| Teraspeed Modeling Services.
| http://www.teraspeed.com
[IBIS Ver]   3.2
[Comment Char] |_char
[File Name]   lpc1788fet208.ibs
[File Rev]   3.0
[Source]  Measured and created by Teraspeed Consulting Group LLC
[Date]   04-04-2011
[Notes]   Quality Check of this IBIS model: Model Passes IBIS Check
   Model parses into ICX IS. Simulation done with Hyperlynx.
   1. MIN TYP MAX information is based on Temperature and Voltage
   characteristics only.
   2. Package data measured using Tektronix IConnect Software.
[Disclaimer]
| NXP Semiconductors warrants and represents that the IBIS models
| identified herein are owned by NXP Semiconductors (NXP).  The
| models provided are not warranted as fully representing all of the
| operating characteristics and specifications of the semiconductor
| products to which the models relate.  Moreover, unless there is a
| signed, written agreement to the contrary, these models are furnished
| on an "as is" basis without support or warranty of any kind, either
| expressed or implied, regarding the use thereof, and NXP
| specifically disclaims all implied warranties of merchantability and
| fitness of the models for any purpose.
| NXP does not assume any liability arising out of the application
| or use of these IBIS models including infringement of patents and
| copyrights, nor does NXP convey any license under its patents and
| copyrights or the rights of others.
| NXP provides IBIS models as a service to our customers.  You and
| your company shall not distribute, convey, sell, or give these models
| to anyone else without receiving prior written permission from
| NXP.
[Copyright]  NXP Semiconductors 2011. All rights reserved.
|   LPC177x_8x (208 TFBGA package) IBIS Model
|   IBIS Model Created by Teraspeed Consulting Group
|   www.teraspeed.com
[Component] LPC1788FET208
[Manufacturer] NXP Semiconductors
[Package]
| variable   typ   min   max
| TFBGA208
R_pkg  1.000E-02  1.000E-02  1.000E-02
L_pkg  2.355E-09  3.067E-10  4.180E-09
C_pkg  5.803E-13  7.558E-14  1.030E-12
[Pin] signal_name  model_name  R_pin  L_pin C_pin
A1   P3_27   io_pad   1.000E-02  4.180E-09  1.030E-12
A2   VSS   GND   1.000E-02  4.180E-09  1.030E-12
A3   P1_0   io_pad   1.000E-02  3.374E-09  8.314E-13
A4   P4_31   io_pad   1.000E-02  3.027E-09  7.458E-13
A5   P1_4   io_pad   1.000E-02  2.726E-09  6.718E-13
A6   P1_9   io_pad   1.000E-02  2.481E-09  6.113E-13
A7   P1_14   io_pad   1.000E-02  2.298E-09  5.663E-13
A8   P1_15   io_pad   1.000E-02  2.185E-09  5.385E-13
A9   P1_17   io_pad   1.000E-02  2.147E-09  5.291E-13
A10   P1_3   io_pad   1.000E-02  2.185E-09  5.385E-13
A11   P4_15   io_pad   1.000E-02  2.298E-09  5.663E-13
A12   VSS   GND   1.000E-02  4.180E-09  1.030E-12
A13   P3_20   io_pad   1.000E-02  2.726E-09  6.718E-13
A14   P1_11   io_pad   1.000E-02  3.027E-09  7.458E-13
A15   P0_8   io_pad   1.000E-02  3.374E-09  8.314E-13
A16   P1_12   io_pad   1.000E-02  3.761E-09  9.267E-13
A17   P1_5   io_pad   1.000E-02  4.180E-09  1.030E-12
B1   P3_2   io_pad   1.000E-02  3.761E-09  9.267E-13
B2   P3_10   io_pad   1.000E-02  3.312E-09  8.162E-13
B3   P3_1   io_pad   1.000E-02  2.895E-09  7.134E-13
B4   P3_0   io_pad   1.000E-02  2.517E-09  6.201E-13
B5   P1_1   io_pad   1.000E-02  2.185E-09  5.385E-13
B6   VSS   GND   1.000E-02  4.180E-09  1.030E-12
B7   P4_30   io_pad   1.000E-02  1.706E-09  4.203E-13
B8   P4_24   io_pad   1.000E-02  1.577E-09  3.887E-13
B9   P4_25   io_pad   1.000E-02  1.534E-09  3.779E-13
B10   P4_29   io_pad   1.000E-02  1.577E-09  3.887E-13
B11   P1_6   io_pad   1.000E-02  1.706E-09  4.203E-13
B12   P0_4   io_pad   1.000E-02  1.911E-09  4.710E-13
B13   Vdd(3v3)   POWER   1.000E-02  4.180E-09  1.030E-12
B14   P3_19   io_pad   1.000E-02  2.517E-09  6.201E-13
B15   P4_14   io_pad   1.000E-02  2.895E-09  7.134E-13
B16   P4_13   io_pad   1.000E-02  3.312E-09  8.162E-13
B17   P2_0   io_pad   1.000E-02  3.761E-09  9.267E-13
C1   P3_13   io_pad   1.000E-02  3.374E-09  8.314E-13
C2   JTAG_TDI   in_pu   1.000E-02  2.895E-09  7.134E-13
C3   P5_4   io_pad   1.000E-02  2.445E-09  6.024E-13
C4   P0_2   io_pad   1.000E-02  2.031E-09  5.004E-13
C5   P3_9   io_pad   1.000E-02  1.663E-09  4.098E-13
C6   P3_22   io_pad   1.000E-02  1.355E-09  3.338E-13
C7   P1_8   io_pad   1.000E-02  1.119E-09  2.758E-13
C8   P1_10   io_pad   1.000E-02  9.710E-10  2.393E-13
C9   Vdd(3v3)   POWER   1.000E-02  4.180E-09  1.030E-12
C10   P3_21   io_pad   1.000E-02  9.710E-10  2.393E-13
C11   P4_28   io_pad   1.000E-02  1.119E-09  2.758E-13
C12   P0_5   io_pad   1.000E-02  1.355E-09  3.338E-13
C13   P0_7   io_pad   1.000E-02  1.663E-09  4.098E-13
C14   P0_9   io_pad   1.000E-02  2.031E-09  5.004E-13
C15   P3_18   io_pad   1.000E-02  2.445E-09  6.024E-13
C16   P4_12   io_pad   1.000E-02  2.895E-09  7.134E-13
C17   Vdd(3v3)   POWER   1.000E-02  4.180E-09  1.030E-12
D1   JTAG_*TRST   in_pu   1.000E-02  3.027E-09  7.458E-13
D2   P3_28   io_pad   1.000E-02  2.517E-09  6.201E-13
D3   JTAG_TDO   tri_pad   1.000E-02  2.031E-09  5.004E-13
D4   P3_12   io_pad   1.000E-02  1.577E-09  3.887E-13
D5   P3_11   io_pad   1.000E-02  1.168E-09  2.877E-13
D6   P0_3   io_pad   1.000E-02  8.165E-10  2.012E-13
D7   Vdd(3v3)   POWER   1.000E-02  4.180E-09  1.030E-12
D8   P3_8   io_pad   1.000E-02  3.675E-10  9.055E-14
D9   P1_2   io_pad   1.000E-02  3.067E-10  7.558E-14
D10   P1_16   io_pad   1.000E-02  3.675E-10  9.055E-14
D11   Vdd(reg)(3v3) POWER   1.000E-02  4.180E-09  1.030E-12
D12   Vss(reg)   GND   1.000E-02  4.180E-09  1.030E-12
D13   P0_6   io_pad   1.000E-02  1.168E-09  2.877E-13
D14   P1_7   io_pad   1.000E-02  1.577E-09  3.887E-13
D15   P2_2   io_pad   1.000E-02  2.031E-09  5.004E-13
D16   P1_13   io_pad   1.000E-02  2.517E-09  6.201E-13
D17   P2_4   io_pad   1.000E-02  3.027E-09  7.458E-13
E1   P0_26   io_pad   1.000E-02  2.726E-09  6.718E-13
E2   JTAG_TCK   in_tck   1.000E-02  2.185E-09  5.385E-13
E3   JTAG_TMS   in_pu   1.000E-02  1.663E-09  4.098E-13
E4   P3_3   io_pad   1.000E-02  1.168E-09  2.877E-13
E14   P2_1   io_pad   1.000E-02  1.168E-09  2.877E-13
E15   VSS   GND   1.000E-02  4.180E-09  1.030E-12
E16   P2_3   io_pad   1.000E-02  2.185E-09  5.385E-13
E17   P2_6   io_pad   1.000E-02  2.726E-09  6.718E-13
F1   P0_25   io_pad   1.000E-02  2.481E-09  6.113E-13
F2   P3_4   io_pad   1.000E-02  1.911E-09  4.710E-13
F3   P3_29   io_pad   1.000E-02  1.355E-09  3.338E-13
F4   P5_0   io_pad   1.000E-02  8.165E-10  2.012E-13
F14   P4_11   io_pad   1.000E-02  8.165E-10  2.012E-13
F15   P3_17   io_pad   1.000E-02  1.355E-09  3.338E-13
F16   P2_5   io_pad   1.000E-02  1.911E-09  4.710E-13
F17   P3_16   io_pad   1.000E-02  2.481E-09  6.113E-13
G1   P3_5   io_pad   1.000E-02  2.298E-09  5.663E-13
G2   P0_24   io_pad   1.000E-02  1.706E-09  4.203E-13
G3   Vdd(3v3)   POWER   1.000E-02  4.180E-09  1.030E-12
G4   Vdda   POWER   1.000E-02  4.180E-09  1.030E-12
G14   P5_3   od1_pad   1.000E-02  5.430E-10  1.338E-13
G15   P4_27   io_pad   1.000E-02  1.119E-09  2.758E-13
G16   P2_7   io_pad   1.000E-02  1.706E-09  4.203E-13
G17   P4_10   io_pad   1.000E-02  2.298E-09  5.663E-13
H1   P0_23   io_pad   1.000E-02  2.185E-09  5.385E-13
H2   P3_14   io_pad   1.000E-02  1.577E-09  3.887E-13
H3   P3_30   io_pad   1.000E-02  9.710E-10  2.393E-13
H4   Vdd(reg)(3v3) POWER   1.000E-02  4.180E-09  1.030E-12
H14   VSS   GND   1.000E-02  4.180E-09  1.030E-12
H15   P2_8   io_pad   1.000E-02  9.710E-10  2.393E-13
H16   P2_9   io_pad   1.000E-02  1.577E-09  3.887E-13
H17   P4_9   io_pad   1.000E-02  2.185E-09  5.385E-13
J1   P3_6   io_pad   1.000E-02  2.147E-09  5.291E-13
J2   Vssa   GND   1.000E-02  4.180E-09  1.030E-12
J3   P3_31   io_pad   1.000E-02  9.202E-10  2.267E-13
J4   P5_1   io_pad   1.000E-02  3.067E-10  7.558E-14
J14   P0_16   io_pad   1.000E-02  3.067E-10  7.558E-14
J15   P4_23   io_pad   1.000E-02  9.202E-10  2.267E-13
J16   P0_15   io_pad   1.000E-02  1.534E-09  3.779E-13
J17   P4_8   io_pad   1.000E-02  2.147E-09  5.291E-13
K1   VREFP   term   1.000E-02  4.180E-09  1.030E-12
K2   RTCX1   term   1.000E-02  1.577E-09  3.887E-13
K3   *RSTOUT   out_pad   1.000E-02  9.710E-10  2.393E-13
K4   Vss(reg)   GND   1.000E-02  4.180E-09  1.030E-12
K14   P4_22   io_pad   1.000E-02  3.675E-10  9.055E-14
K15   P0_18   io_pad   1.000E-02  9.710E-10  2.393E-13
K16   Vdd(3v3)   POWER   1.000E-02  4.180E-09  1.030E-12
K17   P0_17   io_pad   1.000E-02  2.185E-09  5.385E-13
L1   P3_7   io_pad   1.000E-02  2.298E-09  5.663E-13
L2   RTCX2   term   1.000E-02  1.706E-09  4.203E-13
L3   VSS   GND   1.000E-02  4.180E-09  1.030E-12
L4   P2_30   io_pad   1.000E-02  5.430E-10  1.338E-13
L14   P5_2   od1_pad   1.000E-02  5.430E-10  1.338E-13
L15   P4_26   io_pad   1.000E-02  1.119E-09  2.758E-13
L16   P4_7   io_pad   1.000E-02  1.706E-09  4.203E-13
L17   P0_19   io_pad   1.000E-02  2.298E-09  5.663E-13
M1   P3_15   io_pad   1.000E-02  2.481E-09  6.113E-13
M2   *RESET   in_resetb  1.000E-02  1.911E-09  4.710E-13
M3   Vbat   POWER   1.000E-02  4.180E-09  1.030E-12
M4   XTAL1   term   1.000E-02  8.165E-10  2.012E-13
M14   P4_6   io_pad   1.000E-02  8.165E-10  2.012E-13
M15   P4_21   io_pad   1.000E-02  1.355E-09  3.338E-13
M16   P0_21   io_pad   1.000E-02  1.911E-09  4.710E-13
M17   P0_20   io_pad   1.000E-02  2.481E-09  6.113E-13
N1   RTC_ALARM   rtc_alarm  1.000E-02  2.726E-09  6.718E-13
N2   P2_31   io_pad   1.000E-02  2.185E-09  5.385E-13
N3   P2_29   io_pad   1.000E-02  1.663E-09  4.098E-13
N4   XTAL2   term   1.000E-02  1.168E-09  2.877E-13
N14   P2_12   io_pad   1.000E-02  1.168E-09  2.877E-13
N15   P2_10   io_pad   1.000E-02  1.663E-09  4.098E-13
N16   VSS   GND   1.000E-02  4.180E-09  1.030E-12
N17   P0_22   io_pad   1.000E-02  2.726E-09  6.718E-13
P1   P1_31   io_pad   1.000E-02  3.027E-09  7.458E-13
P2   P1_30   io_pad   1.000E-02  2.517E-09  6.201E-13
P3   P2_27   io_pad   1.000E-02  2.031E-09  5.004E-13
P4   P2_28   io_pad   1.000E-02  1.577E-09  3.887E-13
P5   P2_24   io_pad   1.000E-02  1.168E-09  2.877E-13
P6   Vdd(3v3)   POWER   1.000E-02  4.180E-09  1.030E-12
P7   P1_18   io_pad   1.000E-02  5.430E-10  1.338E-13
P8   Vdd(3v3)   POWER   1.000E-02  4.180E-09  1.030E-12
P9   P1_23   io_pad   1.000E-02  3.067E-10  7.558E-14
P10   Vss(reg)   GND   1.000E-02  4.180E-09  1.030E-12
P11   Vdd(reg)(3v3) POWER   1.000E-02  4.180E-09  1.030E-12
P12   VSS   GND   1.000E-02  4.180E-09  1.030E-12
P13   P2_15   io_pad   1.000E-02  1.168E-09  2.877E-13
P14   P4_17   io_pad   1.000E-02  1.577E-09  3.887E-13
P15   P4_18   io_pad   1.000E-02  2.031E-09  5.004E-13
P16   P4_19   io_pad   1.000E-02  2.517E-09  6.201E-13
P17   Vdd(3v3)   POWER   1.000E-02  4.180E-09  1.030E-12
R1   P0_12   io_pad   1.000E-02  3.374E-09  8.314E-13
R2   P0_13   io_pad   1.000E-02  2.895E-09  7.134E-13
R3   P0_28   od2_pad   1.000E-02  2.445E-09  6.024E-13
R4   P2_25   io_pad   1.000E-02  2.031E-09  5.004E-13
R5   P3_24   io_pad   1.000E-02  1.663E-09  4.098E-13
R6   P0_30   io_pad   1.000E-02  1.355E-09  3.338E-13
R7   P2_19   io_pad   1.000E-02  1.119E-09  2.758E-13
R8   P1_21   io_pad   1.000E-02  9.710E-10  2.393E-13
R9   VSS   GND   1.000E-02  4.180E-09  1.030E-12
R10   P1_26   io_pad   1.000E-02  9.710E-10  2.393E-13
R11   P2_16   io_pad   1.000E-02  1.119E-09  2.758E-13
R12   P2_14   io_pad   1.000E-02  1.355E-09  3.338E-13
R13   P2_17   io_pad   1.000E-02  1.663E-09  4.098E-13
R14   P0_11   io_pad   1.000E-02  2.031E-09  5.004E-13
R15   P4_4   io_pad   1.000E-02  2.445E-09  6.024E-13
R16   P4_5   io_pad   1.000E-02  2.895E-09  7.134E-13
R17   P4_20   io_pad   1.000E-02  3.374E-09  8.314E-13
T1   P0_27   od2_pad   1.000E-02  3.761E-09  9.267E-13
T2   P0_31   io_pad   1.000E-02  3.312E-09  8.162E-13
T3   P3_26   io_pad   1.000E-02  2.895E-09  7.134E-13
T4   P2_26   io_pad   1.000E-02  2.517E-09  6.201E-13
T5   VSS   GND   1.000E-02  4.180E-09  1.030E-12
T6   P3_23   io_pad   1.000E-02  1.911E-09  4.710E-13
T7   P0_14   io_pad   1.000E-02  1.706E-09  4.203E-13
T8   P2_20   io_pad   1.000E-02  1.577E-09  3.887E-13
T9   P1_24   io_pad   1.000E-02  1.534E-09  3.779E-13
T10   P1_25   io_pad   1.000E-02  1.577E-09  3.887E-13
T11   P4_2   io_pad   1.000E-02  1.706E-09  4.203E-13
T12   P1_27   io_pad   1.000E-02  1.911E-09  4.710E-13
T13   P1_28   io_pad   1.000E-02  2.185E-09  5.385E-13
T14   P0_1   io_pad   1.000E-02  2.517E-09  6.201E-13
T15   P0_10   io_pad   1.000E-02  2.895E-09  7.134E-13
T16   P2_13   io_pad   1.000E-02  3.312E-09  8.162E-13
T17   P2_11   io_pad   1.000E-02  3.761E-09  9.267E-13
U1   USB_D2N   io_pad   1.000E-02  4.180E-09  1.030E-12
U2   P3_25   io_pad   1.000E-02  3.761E-09  9.267E-13
U3   P2_18   io_pad   1.000E-02  3.374E-09  8.314E-13
U4   P0_29   io_pad   1.000E-02  3.027E-09  7.458E-13
U5   P2_23   io_pad   1.000E-02  2.726E-09  6.718E-13
U6   P1_19   io_pad   1.000E-02  2.481E-09  6.113E-13
U7   P1_20   io_pad   1.000E-02  2.298E-09  5.663E-13
U8   P1_22   io_pad   1.000E-02  2.185E-09  5.385E-13
U9   P4_0   io_pad   1.000E-02  2.147E-09  5.291E-13
U10   P4_1   io_pad   1.000E-02  2.185E-09  5.385E-13
U11   P2_21   io_pad   1.000E-02  2.298E-09  5.663E-13
U12   P2_22   io_pad   1.000E-02  2.481E-09  6.113E-13
U13   Vdd(3v3)   POWER   1.000E-02  4.180E-09  1.030E-12
U14   P1_29   io_pad   1.000E-02  3.027E-09  7.458E-13
U15   P0_0   io_pad   1.000E-02  3.374E-09  8.314E-13
U16   P4_3   io_pad   1.000E-02  3.761E-09  9.267E-13
U17   P4_16   io_pad   1.000E-02  4.180E-09  1.030E-12
[Model Selector]  in_pu
pu_2.5v   input w/int pull up,vdd=2.5v
pu_3.3v   input w/int pull up,vdd=3.3v
[Model Selector]  in_resetb
reset_2.5v   reset input w/int pull up,vdd=2.5v
reset_3.3v   reset input w/int pull up,vdd=3.3v
[Model Selector]  in_tck
tck_2.5v   tck input,vdd=2.5v
tck_3.3v   tck input,vdd=3.3v
[Model Selector]  io_pad
io_2.5v   io pin,vdd=2.5v
io_3.3v   io pin,vdd=3.3v
io_pd_2.5v  io pin w/int pull dwn,vdd=2.5v
io_pd_3.3v  io pin w/int pull dwn,vdd=3.3v
io_pu_2.5v  io pin w/int pull up,vdd=2.5v
io_pu_3.3v  io pin w/int pull up,vdd=3.3v
[Model Selector]  od1_pad
od1_2.5v   open drain1 io pin,vdd=2.5v
od1_3.3v   open drain1 io pin,vdd=3.3v
od1_pd_2.5v  open drain1 io pin w/int pull dwn,vdd=2.5v
od1_pd_3.3v  open drain1 io pin w/int pull dwn,vdd=3.3v
od1_pu_2.5v  open drain1 io pin w/int pull up,vdd=2.5v
od1_pu_3.3v  open drain1 io pin w/int pull up,vdd=3.3v
[Model Selector]  od2_pad
od2_2.5v  open drain2 io pin,vdd=2.5v
od2_3.3v  open drain2 io pin,vdd=3.3v
od2_pd_2.5v  open drain2 io pin w/int pull dwn,vdd=2.5v
od2_pd_3.3v  open drain2 io pin w/int pull dwn,vdd=3.3v
od2_pu_2.5v  open drain2 io pin w/int pull up,vdd=2.5v
od2_pu_3.3v  open drain2 io pin w/int pull up,vdd=3.3v
[Model Selector]  out_pad
out_2.5v   output pin,vdd=2.5v
out_3.3v   output pin,vdd=3.3v
[Model Selector]  tri_pad
tri_2.5v  3-state output pin,vdd=2.5v
tri_3.3v  3-state output pin,vdd=3.3v
[Model] term
Model_type Terminator
C_comp  0pF 0pF 0pF
| variable typ   min   max
[Voltage Range]   3.30000V  3.00000V  3.60000V
[POWER Clamp Reference]  3.30000V  3.00000V  3.60000V
[GND Clamp Reference]   0.00000V  0.00000V  0.00000V
[Temperature Range]   25   85   -40
| Models and submodels in the file (30): pu_2.5v (Input), pu_3.3v (Input), reset_2.5v (Input), reset_3.3v (Input), tck_2.5v (Input), tck_3.3v (Input), io_2.5v (I/O), io_pd_2.5v (I/O), io_pu_2.5v (I/O), io_3.3v (I/O), io_pd_3.3v (I/O), io_pu_3.3v (I/O), od1_2.5v (I/O_open_drain), od1_pd_2.5v (I/O_open_drain), od1_pu_2.5v (I/O_open_drain), od1_3.3v (I/O_open_drain), od1_pd_3.3v (I/O_open_drain), od1_pu_3.3v (I/O_open_drain), od2_2.5v (I/O_open_drain), od2_pd_2.5v (I/O_open_drain), od2_pu_2.5v (I/O_open_drain), od2_3.3v (I/O_open_drain), od2_pd_3.3v (I/O_open_drain), od2_pu_3.3v (I/O_open_drain), out_2.5v (Output), out_3.3v (Output), tri_2.5v (3-state), tri_3.3v (3-state), rtc_alarm (Output), term (Terminator)
